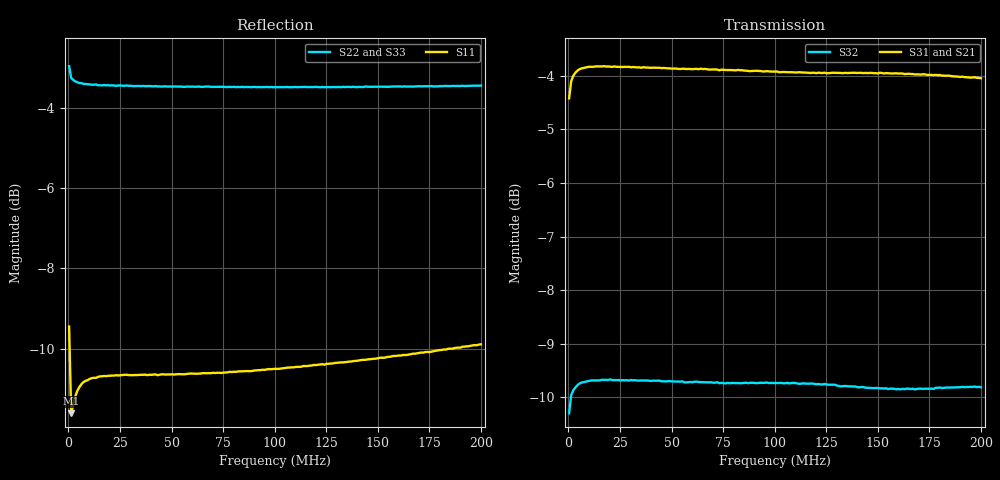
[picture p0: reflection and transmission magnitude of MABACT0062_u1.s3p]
#	MHz	S	RI	R	50
!FREQ	R1	I1	R2	I2	R3	I3
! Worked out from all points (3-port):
!   201 points, 300 kHz to 200 MHz, reference 50 ohm
!   strongest paths, dB at 300 kHz, 50.23 MHz, 100.2 MHz, 150.1 MHz, 200 MHz:
!     S31: -4.4, -3.9, -3.9, -4.0, -4.0
!     S21: -4.5, -3.9, -3.9, -4.1, -4.1
!     S32: -10.3, -9.7, -9.7, -9.8, -9.8
!   lowest |S11| = -11.6 dB at 1.298 MHz (marker M1), VSWR 1.71, Z = 80.3 + j16.4 ohm
!   |S11| at or under -10 dB: 554.3 kHz to 186.2 MHz (185.7 MHz wide, 199 % of centre)
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0.3  0.1543 0.2995  0.5819 0.1515  -0.5815 -0.1528
     0.5763 0.1499  -0.7076 0.0764  -0.2965 -0.0788
     -0.5815 -0.1528  -0.2953 -0.0787  -0.7083 0.0768
1.2985  0.2448 0.0951  0.6215 0.0462  -0.6219 -0.0464
        0.6222 0.0469  -0.6873 0.0262  -0.3173 -0.0242
        -0.6219 -0.0464  -0.3168 -0.0244  -0.687 0.0261
2.297  0.2602 0.0681  0.6296 0.0319  -0.6302 -0.032
       0.6294 0.0323  -0.6838 0.0208  -0.3216 -0.0169
       -0.6302 -0.032  -0.3206 -0.017  -0.683 0.0213
3.2955  0.2701 0.0555  0.6343 0.0255  -0.6345 -0.0256
        0.6336 0.0258  -0.6809 0.0192  -0.3238 -0.0139
        -0.6345 -0.0256  -0.3227 -0.0135  -0.6806 0.0196
6.291  0.2832 0.0367  0.6401 0.0142  -0.6409 -0.0143
       0.6396 0.0141  -0.6776 0.019  -0.3271 -0.00827
       -0.6409 -0.0143  -0.3263 -0.00836  -0.6763 0.0194
18.273  0.2916 0.0191  0.6431 0.000305  -0.6437 0.000488
        0.6429 -0.000214  -0.6729 0.031  -0.3291 -0.00301
        -0.6437 0.000488  -0.3283 -0.00296  -0.6723 0.0328
47.2295  0.2928 0.0199  0.6403 -0.011  -0.6413 0.0128
         0.6398 -0.0121  -0.6681 0.0682  -0.3283 -0.00029
         -0.6413 0.0128  -0.3272 -1.53e-05  -0.6661 0.0727
100.15  0.2964 0.0349  0.6345 -0.0244  -0.6362 0.0287
        0.6348 -0.0252  -0.6556 0.1385  -0.3276 0.00114
        -0.6362 0.0287  -0.3261 0.000702  -0.6509 0.1462
155.0675  0.3046 0.0514  0.6283 -0.0354  -0.6331 0.0413
          0.6225 -0.0373  -0.6375 0.2085  -0.3234 0.000763
          -0.6331 0.0413  -0.3219 0.00159  -0.6281 0.219
200  0.3137 0.064  0.6185 -0.0439  -0.6258 0.0511
     0.6216 -0.0462  -0.6191 0.2642  -0.3253 0.0018
     -0.6258 0.0511  -0.3232 0.00127  -0.6046 0.2742
